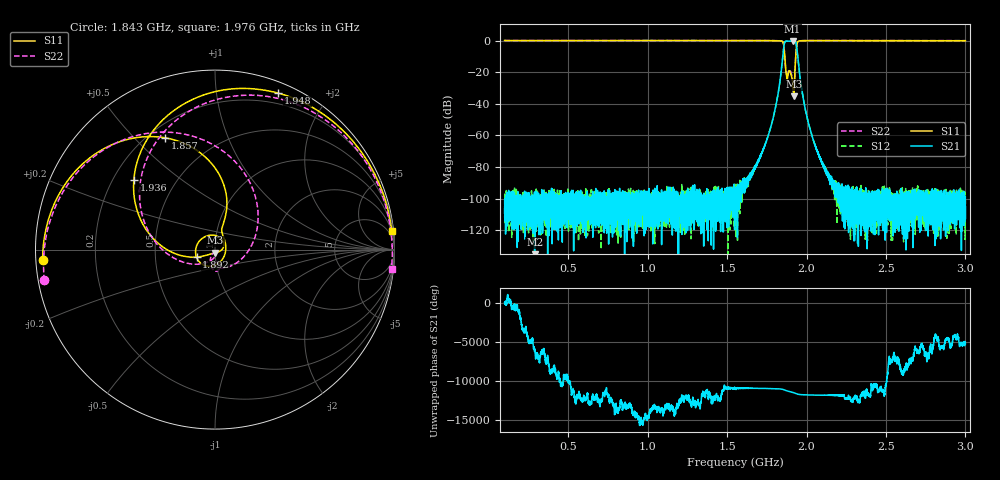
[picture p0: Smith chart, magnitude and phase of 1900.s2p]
# Hz S DB R 50
! Planar, S50180, 20087770, 20.1.2/1
! Date: 23.06.2021 14:48:37
! Data: Format (Calibration Info)
! Freq	S11:dB/Ang(F2)	S21:dB/Ang(F2)	S12:dB/Ang(F2)	S22:dB/Ang(F2)
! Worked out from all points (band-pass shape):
!   8991 points, 100 MHz to 3 GHz, reference 50 ohm
!   highest |S21| = -0.35 dB at 1.912 GHz (marker M1); lowest = -153.5 dB at 289 MHz (marker M2)
!   |S21| within 3 dB of the highest: 1.858 GHz to 1.937 GHz (79.31 MHz wide, 4.18 % of centre)
!   lowest |S11| = -35.3 dB at 1.92 GHz (marker M3), VSWR 1.04, Z = 50.2 - j1.72 ohm
!   |S11| at or under -10 dB: 1.863 GHz to 1.932 GHz (68.9 MHz wide, 3.63 % of centre)
!   |S22| runs from -34.3 to 0.0 dB; largest |S21 - S12| = 0.0024
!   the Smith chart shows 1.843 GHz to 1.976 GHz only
!   S11 on the Smith chart (normalised r, x): 1.843 GHz: 0.02, -0.03; 1.857 GHz: 0.26, +0.62; 1.892 GHz: 0.81, -0.07; 1.936 GHz: 0.29, +0.34; 1.948 GHz: 0.10, +1.47; 1.976 GHz: 2, +19
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1e8  0.02 153.9  -109.16 71.0  -100.37 3.3  0.01 150.1
2.890323e8  -0.03 109.1  -153.53 -137.1  -114.13 99.8  -0.01 100.8
5.835484e8  -0.01 55.3  -100.71 26.0  -97.16 -151.6  0.01 46.0
1.066774e9  -0.00 -4.7  -106.03 29.5  -101.25 152.6  0.04 -10.7
1.55e9  -0.02 -55.6  -100.25 150.3  -96.25 -155.2  0.02 -57.3
1.695806e9  -0.04 -78.6  -76.35 -167.7  -76.02 -164.9  0.02 -77.2
1.801935e9  -0.10 -118.5  -43.78 152.9  -43.79 152.9  -0.03 -112.7
1.826774e9  -0.17 -143.6  -30.08 128.3  -30.08 128.2  -0.09 -135.9
1.843226e9  -0.33 -176.6  -17.36 94.3  -17.36 94.1  -0.30 -169.8
1.857419e9  -3.32 114.1  -3.75 16.3  -3.76 16.2  -3.48 105.6
1.874839e9  -22.70 41.7  -0.40 -119.1  -0.42 -119.1  -21.91 -95.6
1.891935e9  -19.06 -157.2  -0.39 146.4  -0.40 146.3  -18.38 -86.6
1.902258e9  -21.40 110.0  -0.37 92.8  -0.38 92.7  -20.30 -101.9
1.912258e9  -25.77 20.2  -0.35 39.5  -0.36 39.4  -25.66 -118.3
1.92e9  -35.25 -81.4  -0.37 -5.0  -0.38 -5.0  -33.90 -89.8
1.936452e9  -4.50 139.4  -2.82 -130.1  -2.83 -130.2  -4.53 132.9
1.947742e9  -0.54 68.1  -13.03 154.4  -13.03 154.3  -0.54 54.9
1.976129e9  -0.09 6.1  -34.75 91.7  -34.74 91.6  -0.10 -6.1
2.033548e9  -0.05 -32.8  -59.90 54.6  -59.96 53.8  -0.01 -40.7
2.119677e9  -0.04 -55.6  -82.41 30.2  -82.05 37.8  0.02 -60.8
2.516774e9  -0.08 -99.7  -99.63 133.1  -113.92 -177.1  -0.05 -99.8
3e9  -0.13 -136.8  -105.07 179.1  -98.98 29.1  -0.08 -134.1
